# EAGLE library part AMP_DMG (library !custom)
Gameboy Audio Amp. There is no information on this that can be found. All measurements were taken with a caliper with a resolution of 0.01mm/.5mil. Measurements were attempted in both mm and mil. The closest round number was chosen for every dimension, then re-measured for accuracy.
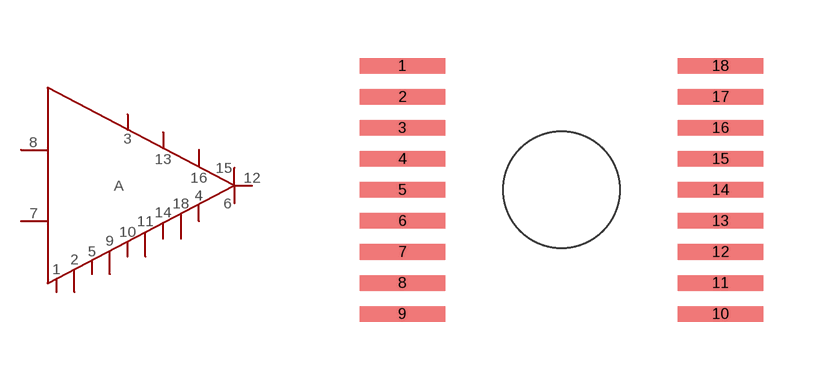
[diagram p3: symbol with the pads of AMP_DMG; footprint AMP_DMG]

Designator prefix A

## AMP_DMG  [AMP_DMG]
1  1  pas
2  2  pas
3  3  pas
4  4  pas
5  5  pas
6  6  pas
7  7  pas
8  8  pas
9  9  pas
10  10  pas
11  11  pas
12  12  pas
13  13  pas
14  14  pas
15  15  pas
16  16  pas
18  18  pas

## Footprint AMP_DMG (pad centres in mm)
smd 2.2 x 0.4: 1 -4.1,3.2; 2 -4.1,2.4; 3 -4.1,1.6; 4 -4.1,0.8; 5 -4.1,0; 6 -4.1,-0.8; 7 -4.1,-1.6; 8 -4.1,-2.4; 9 -4.1,-3.2; 10 4.1,-3.2; 11 4.1,-2.4; 12 4.1,-1.6; 13 4.1,-0.8; 14 4.1,0; 15 4.1,0.8; 16 4.1,1.6; 17 4.1,2.4; 18 4.1,3.2
hole 3 at 0,0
